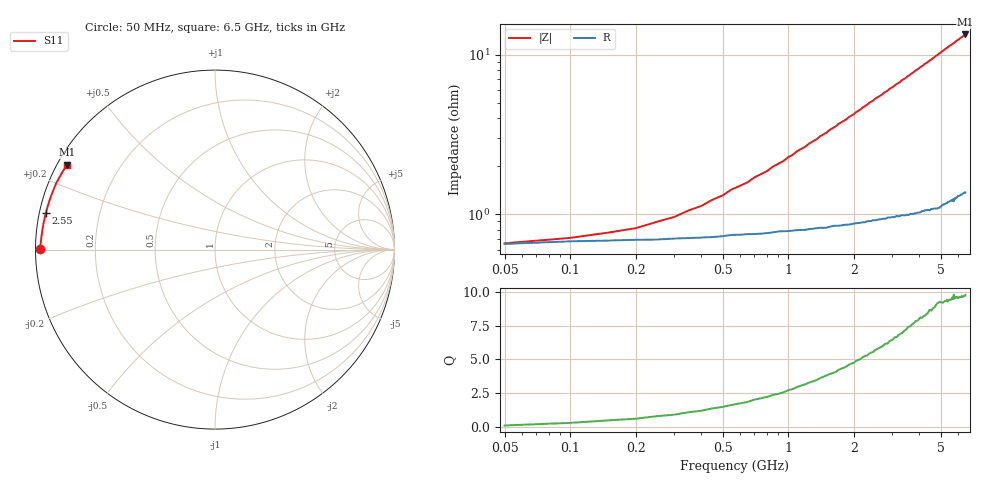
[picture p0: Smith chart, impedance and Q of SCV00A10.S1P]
! Infineon Technologies  Discrete & RF Semiconductors
! BAR63-02L
! Si PIN Diode in TSLP-2
! IF = 100 mA
! S-Parameters:  March  2002
# GHz  S  MA  R  50
!  f  S11
! GHz  MAG  ANG
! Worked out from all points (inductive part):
!   130 points, 50 MHz to 6.5 GHz, reference 50 ohm
!   read as one part to ground: L = 334 pH near 1.15 GHz
!   highest Q = 9.75 at 6.5 GHz (marker M1), where L = 327 pH
!   S11 on the Smith chart (normalised r, x): 50 MHz: 0.01, +0.00; 2.55 GHz: 0.02, +0.11; 6.5 GHz: 0.03, +0.27
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0.05  0.9743 179.8
0.15  0.973 179.2
0.55  0.9708 177.2
0.9  0.9694 175.6
1.7  0.9669 171.8
1.85  0.9664 171.2
1.9  0.9663 170.9
2.45  0.9644 168.4
2.5  0.9644 168.1
2.55  0.9642 167.9
2.7  0.9638 167.3
2.9  0.9631 166.3
3.25  0.9625 164.8
3.3  0.9622 164.5
3.8  0.9612 162.2
4.1  0.9602 160.9
4.35  0.9596 159.8
4.4  0.9597 159.5
4.55  0.9591 158.9
4.9  0.9587 157.2
5.25  0.9566 155.6
5.4  0.9555 155.0
5.45  0.9554 154.7
5.65  0.955 153.9
5.7  0.954 153.6
5.75  0.9554 153.5
5.8  0.9535 153.2
6.5  0.9502 150.1
